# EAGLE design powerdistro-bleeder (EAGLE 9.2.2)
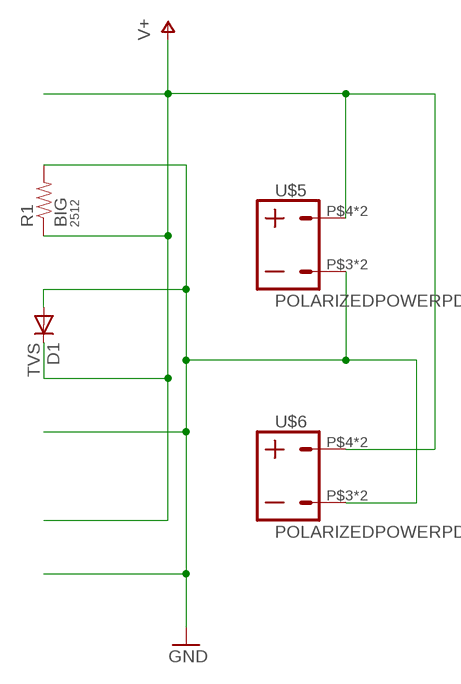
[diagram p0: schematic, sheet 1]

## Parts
D1  TVS  DIODESMA403D  [SMA-403D]
R1  BIG  RESISTOR2512  [R2512]
U$5  POLARIZEDPOWERPDB  [PDBCONN]
U$6  POLARIZEDPOWERPDB  [PDBCONN]

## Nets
GND: D1.P$2(A) R1.2 U$5.P$3 U$5.P$6 U$6.P$3 U$6.P$6
V+: D1.P$1(C) R1.1 U$5.P$4 U$5.P$5 U$6.P$4 U$6.P$5

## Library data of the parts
D1 = passives:DIODE: DIODE
R1 = passives:RESISTOR: Resistor; PACKAGE: 2512
U$5 U$6 = connector:POLARIZEDPOWER

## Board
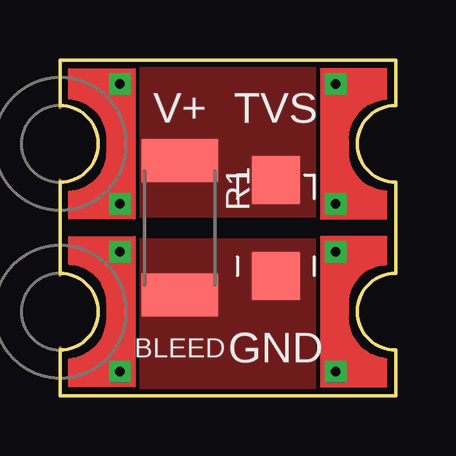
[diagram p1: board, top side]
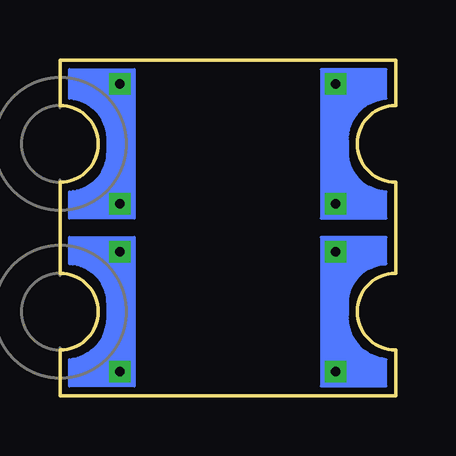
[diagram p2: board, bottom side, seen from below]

Size 14 x 14 mm. Coordinates in mm from the lower left corner, seen from the top.
Outline: 0,5.1 0,8.9 arc90 1.6,10.5 arc90 0,12.1 0,14 14,14 14,12.1 arc90 12.4,10.5 arc90 14,8.9 14,5.1 arc90 12.4,3.5 arc90 14,1.9 14,0 0,0 0,1.9 arc90 1.6,3.5 arc90 0,5.1
Copper layers (1*16): Top 0.035mm / dielectric 1.5mm / Bottom 0.035mm
Design rules "default *": minimum track width 6mil, minimum drill 0.35mm, track to track 6mil, track to pad 6mil, pad to pad 6mil, via to via 6mil, smd to smd 6mil, copper to edge 8mil, drill to drill 6mil, minimum pad ring 10mil, minimum via ring 8mil, stop-mask expansion 4mil, vias tented up to drill 0mil, thermal gap 10mil

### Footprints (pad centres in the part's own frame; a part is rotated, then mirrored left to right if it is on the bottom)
SMA-403D = smd 2 x 2: P$1 -2,0; P$2 2,0
R2512 = smd 1.8 x 3.2: 1 -2.8,0; 2 2.8,0
PDBCONN = drill 0.4 square: P$3 2.5,2.5; P$4 2.5,4.5; P$5 2.5,9.5; P$6 2.5,-2.5

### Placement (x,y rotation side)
D1  9,7 270 top
R1  5,7 270 top
U$5  0,3.5 0 top
U$6  14,3.5 0 bottom

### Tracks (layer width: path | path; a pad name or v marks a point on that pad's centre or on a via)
GND
  pour Top (no thermals): -1,6.5 16.5,6.5 16.5,-0.5 -1,-0.5
  pour Bottom (no thermals): -1.5,6.5 17,6.5 17,-1 -1.5,-1
V+
  pour Top (no thermals): -1,7.5 16.5,7.5 16.5,15 -1,15
  pour Bottom (no thermals): -1.5,7.5 17,7.5 17,15.5 -1.5,15.5

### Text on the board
tPlace: V+ | TVS | BLEED | GND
